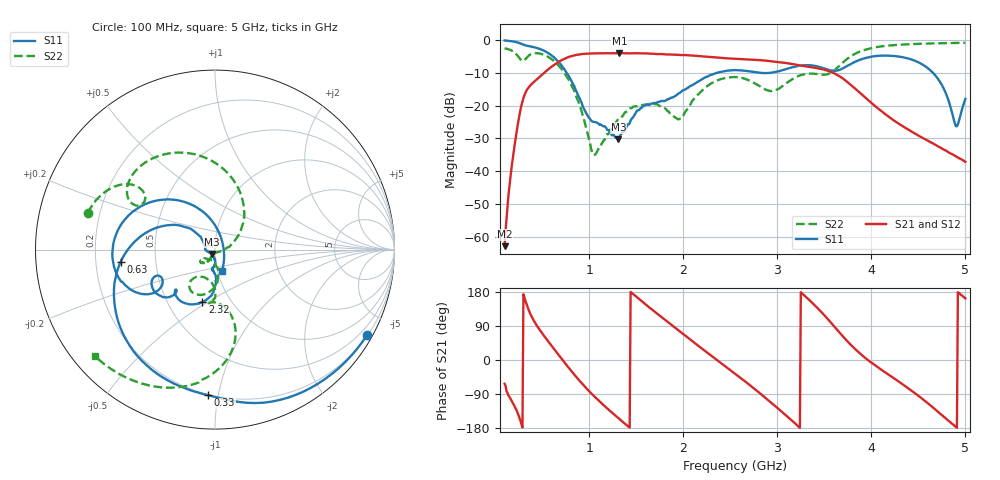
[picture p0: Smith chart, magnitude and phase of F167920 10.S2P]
!  2-Port S-parameters saved by WinCal
! VAR MeasName=S-Parameters (CALIBRATED_DATA) read from VNA (N5242A)
! VAR MeasDate=2016-11-22 9:54:04
! VAR NAME=F167920 10
! VAR FILENAME=F167920 10.S2P
! VAR DATE=2016-11-22 9:54:04
! VAR PHYS_PORTS=1,2
# Hz S DB R 50
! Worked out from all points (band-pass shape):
!   491 points, 100 MHz to 5 GHz, reference 50 ohm
!   highest |S21| = -4.11 dB at 1.32 GHz (marker M1); lowest = -62.7 dB at 100 MHz (marker M2)
!   |S21| within 3 dB of the highest: 653.6 MHz to 3.094 GHz (2.44 GHz wide, 130 % of centre)
!   lowest |S11| = -30.3 dB at 1.31 GHz (marker M3), VSWR 1.06, Z = 48.2 - j2.38 ohm
!   |S11| at or under -10 dB: 758.9 MHz to 2.367 GHz (1.608 GHz wide, 103 % of centre); 2.804 GHz to 2.947 GHz (142.3 MHz wide, 4.95 % of centre); 4.652 GHz to end of sweep
!   |S22| runs from -35.1 to -1.0 dB; largest |S21 - S12| = 0.0013
!   S11 on the Smith chart (normalised r, x): 100 MHz: 0.22, -3.82; 330 MHz: 0.20, -0.94; 630 MHz: 0.31, -0.06; 2.32 GHz: 0.74, -0.47; 5 GHz: 1.05, -0.25
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1e8  -0.25 -29.3  -62.71 -62.7  -62.27 -51.0  -2.65 163.8
2.1e8  -0.67 -61.0  -31.32 -123.9  -31.25 -123.8  -4.01 144.7
3.3e8  -1.81 -92.7  -15.63 149.8  -15.62 149.9  -5.63 151.0
5e8  -3.12 -136.6  -10.60 70.1  -10.59 70.2  -4.44 117.6
6.3e8  -5.51 -172.6  -7.57 27.8  -7.56 27.8  -6.62 86.7
7.7e8  -10.50 153.0  -5.40 -16.9  -5.40 -16.9  -11.65 51.4
9.2e8  -19.26 137.8  -4.37 -61.0  -4.37 -61.1  -21.97 10.7
1.05e9  -24.95 171.7  -4.18 -95.1  -4.19 -95.1  -35.08 -63.5
1.31e9  -30.29 -126.3  -4.14 -153.3  -4.14 -153.3  -24.01 -119.9
1.32e9  -29.66 -118.5  -4.11 -155.5  -4.11 -155.5  -23.91 -121.7
1.74e9  -18.86 -97.1  -4.37 118.9  -4.36 118.9  -19.98 -142.7
1.97e9  -16.02 -87.7  -4.67 74.4  -4.67 74.4  -23.98 -107.6
2.32e9  -10.46 -103.5  -5.34 7.1  -5.34 7.1  -12.94 -94.3
2.55e9  -9.24 -123.1  -5.82 -35.8  -5.82 -35.8  -11.34 -115.4
2.9e9  -10.13 -133.6  -6.44 -105.4  -6.44 -105.5  -15.42 -116.8
3.14e9  -8.53 -134.8  -7.32 -156.5  -7.31 -156.6  -12.35 -89.4
3.37e9  -7.84 -150.2  -8.40 151.2  -8.38 151.1  -10.31 -96.4
3.74e9  -8.05 -144.4  -12.74 50.7  -12.72 50.6  -5.90 -77.2
4.19e9  -4.87 -179.8  -23.51 -39.9  -23.55 -40.1  -1.79 -109.1
4.65e9  -9.93 123.2  -31.38 -124.3  -31.50 -124.4  -1.15 -128.5
4.9e9  -26.27 16.6  -35.42 -176.6  -35.42 -176.9  -1.01 -135.9
5e9  -18.01 -71.6  -37.10 162.7  -37.08 162.2  -0.97 -138.5
